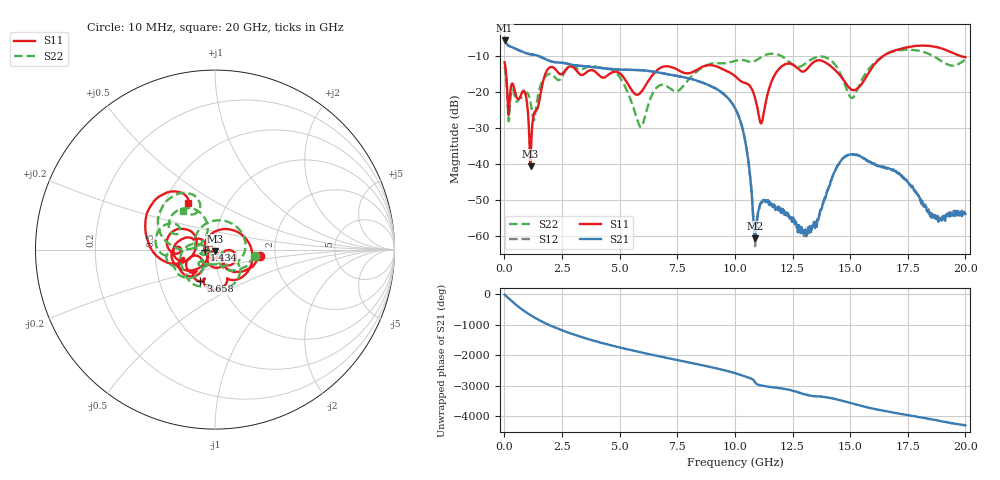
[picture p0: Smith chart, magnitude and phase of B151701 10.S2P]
!  2-Port S-parameters saved by WinCal
! VAR MeasName=S-Parameters (CALIBRATED_DATA) read from VNA (N5244A)
! VAR MeasDate=2015-12-24 19:09:13
! VAR NAME=B151701 10
! VAR FILENAME=B151701 10.S2P
! VAR DATE=2015-12-24 19:09:13
! VAR PHYS_PORTS=1,3
# Hz S DB R 50
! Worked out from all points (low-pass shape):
!   801 points, 10 MHz to 20 GHz, reference 50 ohm
!   highest |S21| = -5.83 dB at 10 MHz (marker M1); lowest = -60.6 dB at 10.88 GHz (marker M2)
!   |S21| within 3 dB of the highest: start of sweep to 740 MHz
!   lowest |S11| = -40.7 dB at 1.134 GHz (marker M3), VSWR 1.02, Z = 50.2 - j0.907 ohm
!   |S11| at or under -10 dB: start of sweep to 16.46 GHz; 19.72 GHz to end of sweep
!   |S22| runs from -29.8 to -8.4 dB; largest |S21 - S12| = 0.0011
!   S11 on the Smith chart (normalised r, x): 10 MHz: 1.67, -0.12; 1.434 GHz: 0.89, -0.00; 3.658 GHz: 0.80, -0.29; 20 GHz: 0.65, +0.37
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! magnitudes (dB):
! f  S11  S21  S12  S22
! 10 MHz  -11.9  -5.8  -5.8  -13.0
! 209.9 MHz  -24.6  -7.4  -7.4  -27.6
! 884.6 MHz  -20.1  -9.2  -9.2  -20.7
! 1.134 GHz  -40.7  -9.7  -9.7  -23.0
! 1.434 GHz  -24.7  -10.0  -10.0  -22.0
! 1.959 GHz  -13.3  -11.5  -11.5  -15.1
! 3.358 GHz  -15.4  -12.9  -12.9  -13.8
! 3.658 GHz  -14.2  -13.1  -13.1  -13.0
! 4.908 GHz  -14.6  -13.8  -13.8  -15.2
! 5.907 GHz  -20.3  -14.1  -14.1  -29.7
! 6.682 GHz  -13.8  -14.7  -14.7  -18.4
! 10.01 GHz  -15.7  -24.6  -24.6  -11.5
! 10.48 GHz  -17.7  -34.8  -34.8  -11.4
! 10.88 GHz  -21.8  -60.6  -62.8  -11.5
! 11.25 GHz  -25.8  -50.0  -50.2  -10.1
! 11.95 GHz  -13.4  -52.6  -52.6  -9.9
! 13.35 GHz  -12.1  -57.2  -57.3  -11.0
! 14.75 GHz  -17.1  -38.2  -38.1  -17.6
! 15.13 GHz  -19.6  -37.3  -37.3  -21.7
! 16.68 GHz  -9.2  -41.2  -41.3  -9.3
! 18.63 GHz  -7.5  -54.5  -54.7  -10.2
! 20 GHz  -10.5  -53.9  -53.6  -11.1
